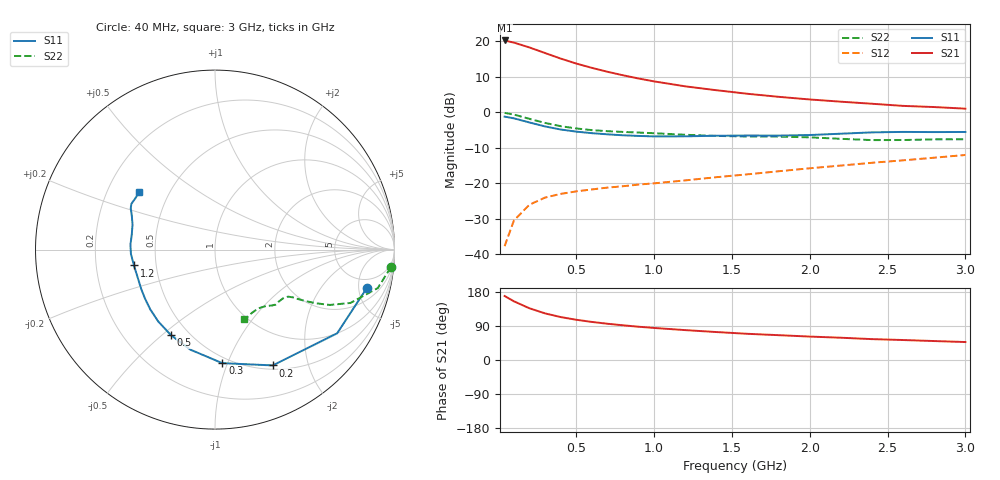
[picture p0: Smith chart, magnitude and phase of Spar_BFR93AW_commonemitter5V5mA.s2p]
! Filename:  BFR93AWA.S2P  Version:  4.0
! NXP part #: BFR93AW  Date: Jun 1994
! Bias condition: Vce=5V, Ic=5mA
#  MHz  S  MA  R  50
! Freq  S11  S21  S12  S22  !GUM [dB]
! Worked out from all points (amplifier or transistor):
!   21 points, 40 MHz to 3 GHz, reference 50 ohm
!   highest |S21| = 20.3 dB at 40 MHz (marker M1)
!   |S21| within 3 dB of that: start of sweep to 265.1 MHz
!   unconditionally stable (mu >= 1): 995.9 MHz to end of sweep
!   at 300 MHz: K = 0.42, MSG = 20.4 dB, |S12| = -24.0 dB
!   at 1 GHz: K = 1.00, MAG = 14.1 dB, |S12| = -20.0 dB
!   at 3 GHz: K = 1.04, MAG = 5.3 dB, |S12| = -12.0 dB
!   lowest NFmin = 1.20 dB at 500 MHz
!   S11 on the Smith chart (normalised r, x): 40 MHz: 3.40, -6.12; 200 MHz: 0.55, -1.47; 300 MHz: 0.45, -0.96; 500 MHz: 0.40, -0.54; 1.2 GHz: 0.37, -0.08; 3 GHz: 0.34, +0.30
40  0.872 -14.3  10.34 168.9  0.013 81.9  0.985 -5.7
100  0.825 -34.4  9.64 154.8  0.03 71.4  0.932 -13.3
200  0.721 -63.5  8.237 136.4  0.05 59.6  0.811 -21.5
300  0.634 -86.3  6.875 123.0  0.063 52.9  0.711 -25.7
400  0.574 -103.9  5.746 113.3  0.071 49.8  0.64 -27.9
500  0.536 -117.3  4.888 106.2  0.077 48.8  0.594 -29.2
600  0.51 -128.4  4.251 100.5  0.082 49.4  0.563 -30.1
700  0.491 -137.2  3.744 95.7  0.087 50.6  0.544 -30.6
800  0.476 -145.0  3.341 91.6  0.091 52.1  0.531 -31.0
900  0.466 -151.9  3.01 87.8  0.096 53.7  0.52 -31.1
1000  0.459 -158.1  2.739 84.6  0.1 55.5  0.509 -31.5
1200  0.46 -168.9  2.333 78.9  0.11 59.2  0.484 -32.8
1400  0.469 -177.0  2.057 73.8  0.122 62.6  0.466 -35.7
1600  0.472 176.5  1.832 69.1  0.134 65.4  0.458 -39.5
1800  0.471 170.1  1.659 65.5  0.148 68.3  0.456 -42.2
2000  0.48 163.2  1.523 61.8  0.163 70.9  0.445 -44.4
2200  0.501 157.7  1.417 58.8  0.178 72.8  0.424 -47.8
2400  0.523 153.9  1.325 55.1  0.195 74.3  0.407 -53.5
2600  0.531 151.3  1.236 52.7  0.211 75.0  0.408 -59.8
2800  0.528 147.5  1.19 50.0  0.23 76.1  0.417 -64.2
3000  0.53 142.6  1.13 47.4  0.251 76.7  0.418 -67.2
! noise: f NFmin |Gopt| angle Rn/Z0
500  1.2  0.22  61.3  0.168
1000  1.9  0.25  142.8  0.23
2000  3  0.71  -154.5  0.1
